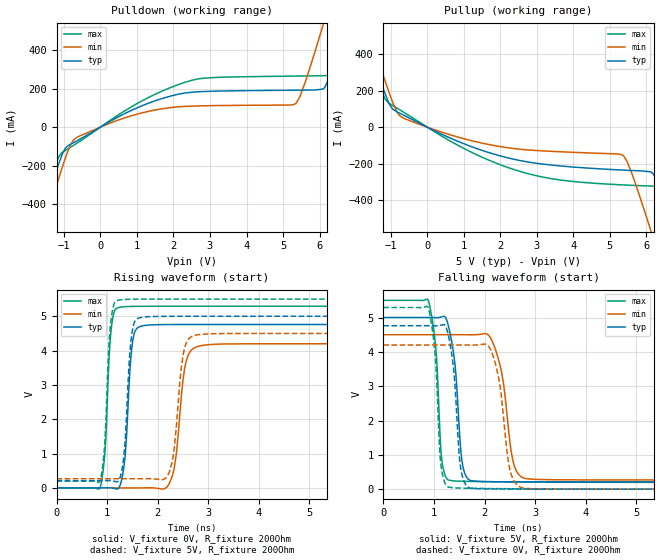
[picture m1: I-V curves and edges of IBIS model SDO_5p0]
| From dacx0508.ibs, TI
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|   Model
[Model]   SDO_5p0
Model_type   Output
Polarity   Non-Inverting
Vmeas = 2.5
Vref = 0
Cref = 1pF
Rref = 100000
|   typ   min   max
C_comp   1.9754pF   1.62052pF   2.35317pF
| Where nom  PVT is Nominal Process, 5.0V, 27C
|   Fast PVT is Strong Process,  5.5V, -40C
|   Slow PVT is Weak Process,   4.5V, 125C
[Voltage Range]   5   4.5   5.5
|Junction Temperature
[Temperature Range]   27   125   -40
[Pullup Reference]   5   4.5   5.5
[Pulldown Reference]   0   0   0
[Power Clamp Reference]   5   4.5   5.5
[GND Clamp Reference]   0   0   0
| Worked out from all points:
|   slope of the pulldown table from 0 to 0.75 V, typ, clamps not added: 9.61 ohm
|   slope of the pullup table from 0 to 0.75 V, typ, clamps not added: 10.7 ohm
|   falling waveform, V_fixture 5V, R_fixture 200Ohm: 20-80 % time 149ps typ, 227ps min, 119ps max; typ from 5 V to 0.211 V
|   rising waveform, V_fixture 0V, R_fixture 200Ohm: 20-80 % time 112ps typ, 167ps min, 100ps max; typ from 0 V to 4.76 V
|   rising waveform, V_fixture 5V, R_fixture 200Ohm: 20-80 % time 111ps typ, 156ps min, 96.4ps max; typ from 0.211 V to 5 V
|   falling waveform, V_fixture 0V, R_fixture 200Ohm: 20-80 % time 139ps typ, 206ps min, 114ps max; typ from 4.76 V to 0 V
[Pulldown]
|   Voltage   I(typ)   I(min)   I(max)
-5V       -2.704A    -2.779A    -2.658A
-2.195V   -855.7mA   -935.1mA   -805.9mA
-1.58V    -458.8mA   -539.1mA   -408.2mA
-1.145V   -193.2mA   -268.4mA   -155.8mA
-725mV    -79.65mA   -64.21mA   -93.36mA
640mV     67.98mA    46.69mA    81.52mA
2.65V     183.4mA    110.1mA    249.6mA
5.335V    191.9mA    120.8mA    265.3mA
6.1V      198.3mA    533.1mA    267.3mA
6.805V    589.9mA    986.3mA    275.3mA
7.27V     890.2mA    1.289A     522.8mA
10V       2.688A     3.088A     2.314A
[Pullup]
|   Voltage   I(typ)   I(min)   I(max)
-5V       2.688A     2.757A     2.645A
-2.15V    810.1mA    884.5mA    764mA
-1.73V    538.5mA    613.7mA    491.9mA
-1.655V   490.6mA    565.7mA    443.9mA
-1.16V    187.2mA    257.5mA    156mA
-755mV    76.9mA     62.84mA    95.4mA
2.245V    -170.6mA   -114.3mA   -224.3mA
5.35V     -235.8mA   -153.8mA   -317.2mA
6.1V      -245mA     -555.8mA   -323.4mA
6.865V    -646.4mA   -1.048A    -338.7mA
7.3V      -927.2mA   -1.331A    -557.5mA
10V       -2.705A    -3.11A     -2.328A
[Ramp]
R_load = 200
|   typ   min   max
dV/dt_r   2.85629/1.11775e-10   2.51978/1.67498e-10   3.17481/1.00389e-10
dV/dt_f   2.87354/1.49374e-10   2.53929/2.27194e-10   3.18142/1.19398e-10
[Falling Waveform]
V_fixture = 5V
V_fixture_min = 4.5V
V_fixture_max = 5.5V
R_fixture = 200Ohm
C_fixture = 0F
|   Time   V(typ)   V(min)   V(max)
0s        5V         4.5V       5.5V
880.1ps   5V         4.5V       5.521V
1.037ns   4.997V     4.5V       4.086V
1.153ns   5.02V      4.5V       881.8mV
1.317ns   4.547V     4.5V       255.7mV
1.555ns   801.4mV    4.5V       229.4mV
1.767ns   241.5mV    4.497V     224.1mV
2.181ns   217mV      4.205V     215.8mV
2.852ns   213.6mV    301.8mV    207.9mV
20ns      210.7mV    267.8mV    197.6mV
[Rising Waveform]
V_fixture = 0V
V_fixture_min = 0V
V_fixture_max = 0V
R_fixture = 200Ohm
C_fixture = 0F
|   Time   V(typ)   V(min)   V(max)
0s        19.62uV    26.57uV    14.41uV
861.1ps   -180.9uV   -40.74uV   7.327mV
1.087ns   861.4uV    -58.37uV   4.697V
1.275ns   167.7mV    -73.07uV   5.267V
1.511ns   4.328V     -91.53uV   5.286V
1.712ns   4.724V     1.13mV     5.288V
2.225ns   4.758V     113.5mV    5.291V
2.562ns   4.759V     3.688V     5.291V
2.929ns   4.759V     4.16V      5.291V
20ns      4.761V     4.2V       5.291V
[Rising Waveform]
V_fixture = 5V
V_fixture_min = 4.5V
V_fixture_max = 5.5V
R_fixture = 200Ohm
C_fixture = 0F
|   Time   V(typ)   V(min)   V(max)
0s        210.7mV    267.8mV    197.6mV
861.1ps   210.6mV    267.8mV    206.8mV
1.069ns   213.7mV    267.8mV    4.778V
1.236ns   229.2mV    267.8mV    5.471V
1.49ns    4.509V     267.8mV    5.496V
1.666ns   4.963V     268mV      5.498V
2.225ns   4.997V     442.6mV    5.499V
2.502ns   4.999V     3.87V      5.499V
2.783ns   4.999V     4.458V     5.499V
20ns      5V         4.5V       5.5V
[Falling Waveform]
|Gnd
V_fixture = 0V
V_fixture_min = 0V
V_fixture_max = 0V
R_fixture = 200Ohm
C_fixture = 0F
|   Time   V(typ)   V(min)   V(max)
0s        4.761V     4.2V       5.291V
880.1ps   4.761V     4.2V       5.311V
1.137ns   4.775V     4.2V       709.1mV
1.317ns   4.241V     4.2V       52.06mV
1.533ns   562.4mV    4.2V       31.34mV
1.712ns   31.19mV    4.198V     25.67mV
2.143ns   5.842mV    3.982V     17.63mV
2.502ns   2.991mV    560mV      13.5mV
2.783ns   2.259mV    25.26mV    10.82mV
20ns      19.87uV    27.03uV    14.9uV
